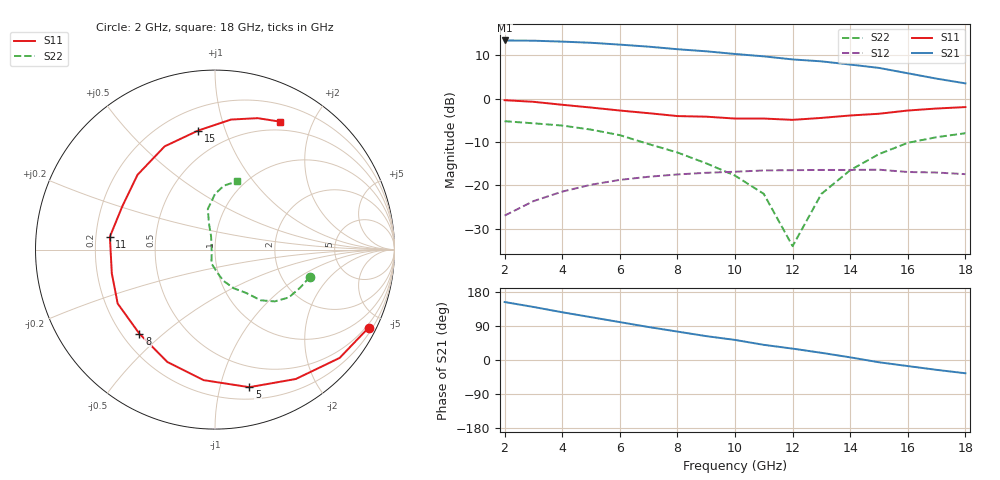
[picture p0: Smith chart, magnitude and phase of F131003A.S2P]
!ATF-13100
!S-PARAMETERS at Vds=2.5V  Id=20mA.  LAST UPDATED 07-22-92
# ghz s ma r 50
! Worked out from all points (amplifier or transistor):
!   17 points, 2 GHz to 18 GHz, reference 50 ohm
!   highest |S21| = 13.4 dB at 2 GHz (marker M1)
!   |S21| within 3 dB of that: start of sweep to 9.815 GHz
!   unconditionally stable (mu >= 1): 11.97 GHz to end of sweep
!   at 4 GHz: K = 0.42, MSG = 17.3 dB, |S12| = -21.4 dB
!   at 10 GHz: K = 0.86, MSG = 13.6 dB, |S12| = -16.8 dB
!   at 18 GHz: K = 1.10, MAG = 8.5 dB, |S12| = -17.4 dB
!   lowest NFmin = 0.70 dB at 6 GHz
!   S11 on the Smith chart (normalised r, x): 2 GHz: 0.37, -4.13; 5 GHz: 0.30, -1.23; 8 GHz: 0.27, -0.42; 11 GHz: 0.26, +0.06; 15 GHz: 0.34, +0.81; 18 GHz: 0.39, +1.56
2  0.96 -27.0  4.68 153.0  0.045 75.0  0.55 -16.0
3  0.92 -41.0  4.65 140.0  0.066 67.0  0.52 -24.0
4  0.85 -58.0  4.54 126.0  0.085 59.0  0.49 -33.0
5  0.79 -76.0  4.4 113.0  0.102 50.0  0.44 -41.0
6  0.73 -95.0  4.19 100.0  0.116 42.0  0.38 -48.0
7  0.68 -113.0  3.97 87.0  0.126 34.0  0.3 -54.0
8  0.63 -132.0  3.71 75.0  0.134 25.0  0.24 -64.0
9  0.62 -151.0  3.51 63.0  0.14 18.0  0.18 -75.0
10  0.59 -167.0  3.27 53.0  0.144 11.0  0.13 -84.0
11  0.59 173.0  3.07 40.0  0.149 2.0  0.08 -104.0
12  0.57 155.0  2.83 30.0  0.15 -9.0  0.02 160.0
13  0.6 136.0  2.69 19.0  0.151 -16.0  0.08 106.0
14  0.64 116.0  2.47 7.0  0.151 -25.0  0.15 103.0
15  0.67 98.0  2.26 -6.0  0.152 -34.0  0.23 100.0
16  0.73 83.0  1.96 -16.0  0.143 -40.0  0.31 90.0
17  0.77 72.0  1.7 -26.0  0.141 -45.0  0.36 82.0
18  0.8 63.0  1.5 -35.0  0.135 -48.0  0.4 72.0
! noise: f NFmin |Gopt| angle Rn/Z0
6  0.7  0.32  68  0.21
8  0.8  0.25  102  0.15
12  1.1  0.23  165  0.09
15  1.5  0.32  -112  0.21
